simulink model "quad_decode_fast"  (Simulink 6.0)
settings: Solver=ode45  StartTime=0.0  StopTime=tmax  RelTol=1e-3
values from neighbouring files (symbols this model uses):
  deltat = .001    (= 0.001)    [run_quad_decode.m]

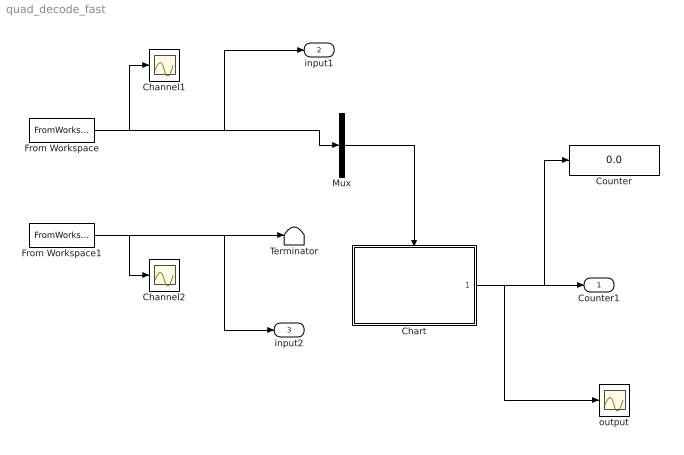
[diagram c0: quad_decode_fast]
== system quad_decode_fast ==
  Channel1 : Scope
  Channel2 : Scope
  Chart : Stateflow chart  TreatAsAtomicUnit=on
  Counter : Display
  From Workspace : FromWorkspace  VariableName=fqd1  SampleTime=deltat
  From Workspace1 : FromWorkspace  VariableName=fqd2  SampleTime=deltat
  Mux : Mux  Inputs=1
  Terminator : Terminator
  output : Scope
  Counter1 : Outport
  input1 : Outport  Port=2
  input2 : Outport  Port=3
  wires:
  From Workspace/1 -> Channel1/1, Mux/1, input1/1
  Chart/1(counter) -> output/1, Counter1/1, Counter/1
  From Workspace1/1 -> Channel2/1, Terminator/1, input2/1
  Mux/1 -> Chart/Trigger

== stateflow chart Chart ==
  state state0
  (default) -> state0
  state0 -> (junction 4) : primary{counter=counter+4;}
  (junction 4) -> state0
